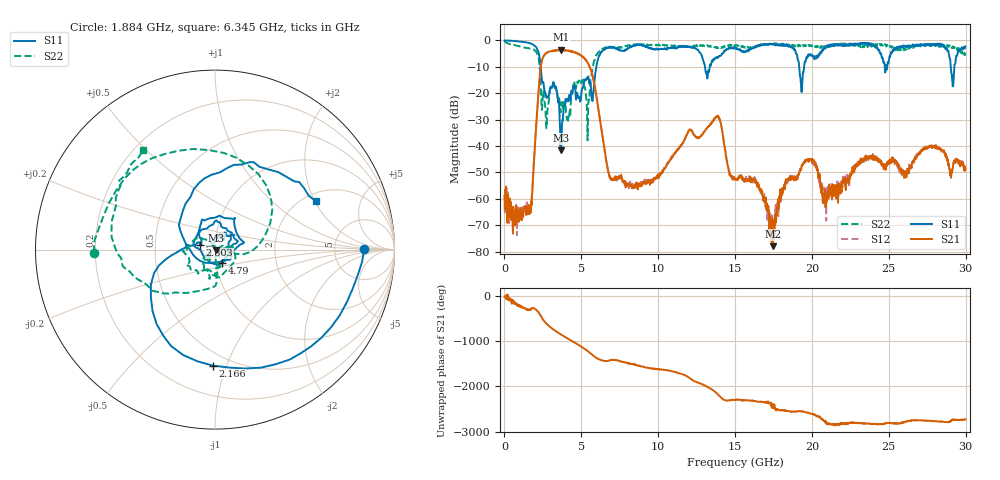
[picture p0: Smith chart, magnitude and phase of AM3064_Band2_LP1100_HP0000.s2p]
# Hz S DB R 50.0
!freq dBS11 angS11 dBS21 angS21 dBS12 angS12 dBS22 angS22
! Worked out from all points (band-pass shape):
!   1600 points, 10 MHz to 29.98 GHz, reference 50 ohm
!   highest |S21| = -3.54 dB at 3.703 GHz (marker M1); lowest = -77.9 dB at 17.46 GHz (marker M2)
!   |S21| within 3 dB of the highest: 2.502 GHz to 5.14 GHz (2.638 GHz wide, 69 % of centre); 5.159015 GHz to 5.167312 GHz (8.298 MHz wide, 0.161 % of centre)
!   lowest |S11| = -41.5 dB at 3.684 GHz (marker M3), VSWR 1.02, Z = 50.7 - j0.506 ohm
!   |S11| at or under -10 dB: 2.357 GHz to 5.982 GHz (3.625 GHz wide, 86.9 % of centre); 13.04 GHz to 13.35 GHz (305.9 MHz wide, 2.32 % of centre); 19.17 GHz to 19.49 GHz (325.7 MHz wide, 1.68 % of centre)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
!   |S22| runs from -37.8 to -0.3 dB; largest |S21 - S12| = 0.022
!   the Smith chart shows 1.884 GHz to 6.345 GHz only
!   S11 on the Smith chart (normalised r, x): 1.884 GHz: 11, +0; 2.166 GHz: 0.40, -0.89; 2.803 GHz: 0.85, +0.05; 4.79 GHz: 1.07, -0.16; 6.345 GHz: 2.31, +2.03
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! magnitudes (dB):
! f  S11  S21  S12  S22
! 10 MHz  0.0  -58.9  -58.2  -0.3
! 1.566 GHz  -1.0  -62.3  -63.6  -2.9
! 1.884 GHz  -1.6  -48.5  -49.0  -3.4
! 2.166 GHz  -3.8  -23.5  -23.5  -5.6
! 2.803 GHz  -21.3  -4.5  -4.5  -26.2
! 3.684 GHz  -41.5  -3.8  -3.6  -23.9
! 3.703 GHz  -39.6  -3.5  -3.8  -23.7
! 4.79 GHz  -21.7  -5.1  -4.9  -15.9
! 5.015 GHz  -19.2  -5.8  -5.9  -16.3
! 5.427 GHz  -14.0  -8.7  -8.5  -31.1
! 6.345 GHz  -4.1  -35.1  -35.0  -3.3
! 6.964 GHz  -2.5  -52.3  -52.2  -2.7
! 10 GHz  -3.4  -50.7  -51.4  -1.8
! 13.82 GHz  -6.4  -28.7  -28.8  -2.5
! 15 GHz  -2.8  -52.8  -52.5  -1.8
! 16.34 GHz  -2.5  -54.0  -53.6  -2.5
! 17.46 GHz  -1.4  -77.9  -69.7  -1.3
! 19.32 GHz  -19.4  -47.9  -47.4  -1.9
! 19.99 GHz  -5.4  -45.4  -45.4  -1.9
! 20.85 GHz  -2.9  -56.5  -57.8  -2.5
! 25 GHz  -7.9  -46.2  -45.9  -1.8
! 29.98 GHz  -2.3  -48.5  -49.1  -4.7
